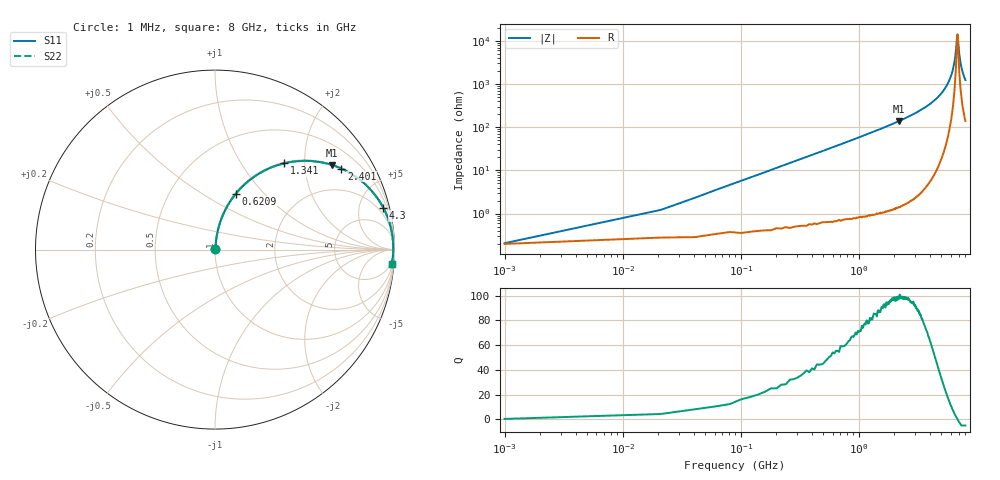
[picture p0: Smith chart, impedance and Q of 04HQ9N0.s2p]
! Coilcraft 0403HQ-9N0 Chip Inductor
! 13 February 2004
# MHZ S MA R 50
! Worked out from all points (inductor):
!   401 points, 1 MHz to 8 GHz, reference 50 ohm
!   read as one part in series: L = 9.03 nH near 40.99 MHz
!   highest Q = 98.9 at 2.181 GHz (marker M1), where L = 10 nH
!   self-resonance near 6.84 GHz
!   S11 on the Smith chart (normalised r, x): 1 MHz: 1.00, +0.00; 620.9 MHz: 1.01, +0.71; 1.341 GHz: 1.02, +1.58; 2.401 GHz: 1.03, +3.10; 4.3 GHz: 1.15, +8.02; 8 GHz: 4, -25
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1  0.002027 16.1  0.998 -0.0  0.998 -0.0  0.002027 16.1
60.992  0.035 82.6  0.996 -2.0  0.996 -2.0  0.035 82.6
100.988  0.057 83.1  0.995 -3.3  0.995 -3.3  0.057 83.1
140.982  0.079 82.6  0.993 -4.5  0.993 -4.5  0.079 82.6
320.96  0.178 78.1  0.979 -10.3  0.979 -10.3  0.178 78.1
620.922  0.332 69.6  0.937 -19.4  0.937 -19.4  0.332 69.6
1340.832  0.616 51.3  0.781 -38.0  0.781 -38.0  0.616 51.3
2180.727  0.804 35.9  0.586 -53.5  0.586 -53.5  0.804 35.9
2400.7  0.836 32.7  0.54 -56.7  0.54 -56.7  0.836 32.7
2680.665  0.869 29.0  0.486 -60.4  0.486 -60.4  0.869 29.0
4000.5  0.956 16.2  0.278 -72.9  0.278 -72.9  0.956 16.2
4300.462  0.966 13.9  0.241 -75.0  0.241 -75.0  0.966 13.9
5340.333  0.987 7.4  0.128 -80.3  0.128 -80.3  0.987 7.4
6180.228  0.992 3.0  0.053 -80.4  0.053 -80.4  0.992 3.0
6500.188  0.993 1.5  0.028 -74.8  0.028 -74.8  0.993 1.5
6680.165  0.993 0.7  0.015 -61.5  0.015 -61.5  0.993 0.7
6800.15  0.993 0.2  0.007942 -28.4  0.007942 -28.4  0.993 0.2
6860.143  0.993 -0.0  0.007099 5.6  0.007099 5.6  0.993 -0.0
7080.115  0.992 -1.0  0.018 65.3  0.018 65.3  0.992 -1.0
7300.088  0.992 -1.9  0.033 74.7  0.033 74.7  0.992 -1.9
7580.053  0.99 -3.0  0.052 78.0  0.052 78.0  0.99 -3.0
8000  0.988 -4.6  0.08 79.0  0.08 79.0  0.988 -4.6
